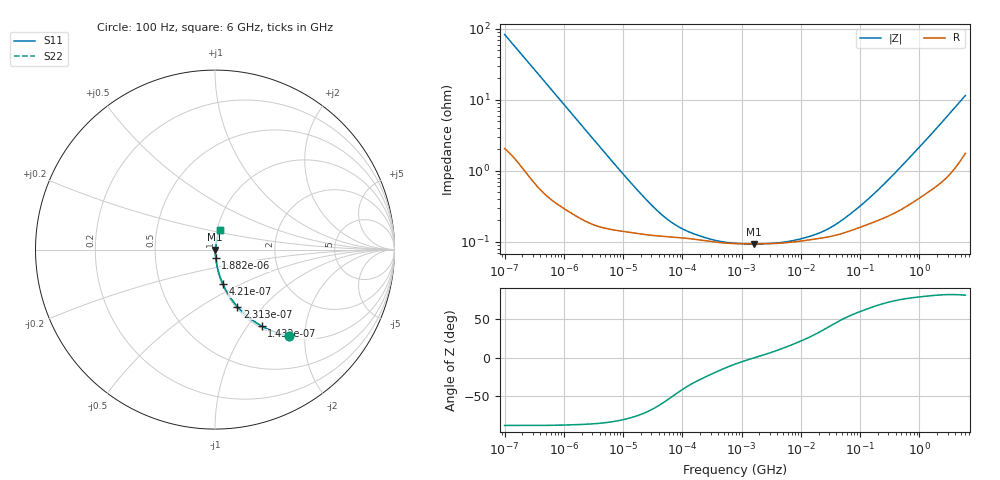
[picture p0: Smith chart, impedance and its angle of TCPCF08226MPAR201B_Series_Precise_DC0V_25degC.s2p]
! TCPCF08226MPAR201B Polymer Tantalum Capacitor Sparameter Model
! Model Generated by Samsung Electro-Mechanics
! Samsung Sparameter Version 5.0
! Date : Oct-21-2025
! Products : Polymer Tantalum Capacitor
! Characteristics :
!  Nominal Capacitance = 22uF
!  Capacitance Tolerance = +/-20%
!  ESR = 200 mohm max at 100kHz
!  Rated Voltage = 8Vdc
!  Size = 0805(unit:inch), 2012(unit:mm)
!  Length = 2.00+/-0.20mm
!  Width = 1.25+/-0.20mm
!  Thickness = 0.55+/-0.10mm
!  Lineup = Conductive Polymer Type
!  Feature = PCF
!  Measurement Temperature : 25degC.
!  DC bias Value = 0V
!  Frequency : 100Hz ~ 6GHz
! External Node Assignments :
!  1  o---||---o  2
# MHz S RI R 50.0
! Freq.  Real(S11)  Im(S11)  Real(S12)  Im(S12)  Real(S21)  Im(S21)  Real(S22)  Im(S22)
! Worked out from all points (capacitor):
!   300 points, 100 Hz to 6 GHz, reference 50 ohm
!   read as one part in series: C = 19 uF near 106.2 Hz
!   lowest |Z| = 92.9 mohm at 1.638 MHz (marker M1)
!   series resonance near 1.699 MHz, so ESL is about 460 pH
!   S11 on the Smith chart (normalised r, x): 100 Hz: 1.04, -1.67; 143.2 Hz: 1.03, -1.17; 231.3 Hz: 1.02, -0.73; 421 Hz: 1.01, -0.41; 1.882 kHz: 1.00, -0.09; 6 GHz: 1.04, +0.23
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0.0001  0.4117 -0.4799  0.5883 0.4799  0.5883 0.4799  0.4117 -0.4799
0.0001432463  0.261 -0.4263  0.739 0.4263  0.739 0.4263  0.261 -0.4263
0.00023131  0.1244 -0.3175  0.8756 0.3175  0.8756 0.3175  0.1244 -0.3175
0.0004210496  0.044 -0.1926  0.956 0.1926  0.956 0.1926  0.044 -0.1926
0.0008137405  0.0142 -0.1037  0.9858 0.1037  0.9858 0.1037  0.0142 -0.1037
0.001882263  0.00424 -0.0459  0.9958 0.0459  0.9958 0.0459  0.00424 -0.0459
0.001998454  0.00394 -0.0432  0.9961 0.0432  0.9961 0.0432  0.00394 -0.0432
0.01358747  0.00139 -0.00657  0.9986 0.00657  0.9986 0.00657  0.00139 -0.00657
0.03993819  0.00121 -0.00232  0.9988 0.00232  0.9988 0.00232  0.00121 -0.00232
0.0726988  0.00116 -0.00133  0.9988 0.00133  0.9988 0.00133  0.00116 -0.00133
0.1323324  0.0011 -0.000798  0.9989 0.000798  0.9989 0.000798  0.0011 -0.000798
0.3450549  0.000988 -0.000359  0.999 0.000359  0.999 0.000359  0.000988 -0.000359
0.7981464  0.000937 -0.000136  0.9991 0.000136  0.9991 0.000136  0.000937 -0.000136
1.637756  0.000928 -6e-06  0.9991 6e-06  0.9991 6e-06  0.000928 -6e-06
5.426588  0.000963 0.000225  0.999 -0.000225  0.999 -0.000225  0.000963 0.000225
15.95059  0.00108 0.000586  0.9989 -0.000586  0.9989 -0.000586  0.00108 0.000586
29.03458  0.00117 0.000966  0.9988 -0.000966  0.9988 -0.000966  0.00117 0.000966
56.11362  0.00134 0.00169  0.9987 -0.00169  0.9987 -0.00169  0.00134 0.00169
137.8087  0.00177 0.00358  0.9982 -0.00358  0.9982 -0.00358  0.00177 0.00358
318.7652  0.0024 0.00744  0.9976 -0.00744  0.9976 -0.00744  0.0024 0.00744
1922.593  0.0074 0.038  0.9926 -0.038  0.9926 -0.038  0.0074 0.038
6000  0.0294 0.1083  0.9706 -0.1083  0.9706 -0.1083  0.0294 0.1083
